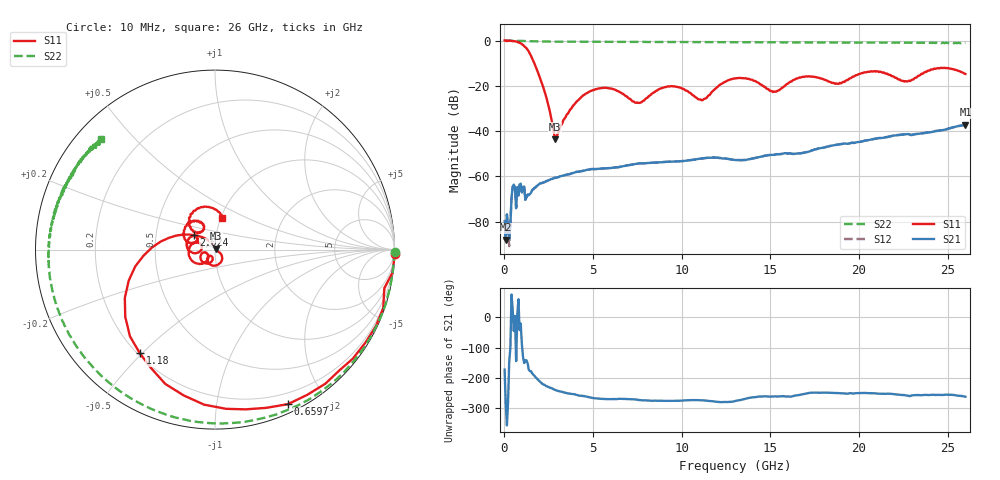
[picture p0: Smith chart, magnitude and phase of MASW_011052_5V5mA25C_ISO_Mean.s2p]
! MA-COM, USA
! Part Number: MASW-011052
! Data: 29-03-2013
! Bias Condition:
!  Isolation in OFF stage Antenna (1) to RFin (2)
!  Forward Bias (series Diode and Shunt Diode) I = 5 mA
!  Reverse Bias Voltage V = -5V
!  Temp: 25C
!  VAR RecID: Mean
# HZ S DB R 50
! F n11x n11y n21x n21y n12x n12y n22x n22y
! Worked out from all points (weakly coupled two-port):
!   401 points, 10 MHz to 26 GHz, reference 50 ohm
!   highest |S21| = -37.23 dB at 26 GHz (marker M1); lowest = -88.0 dB at 74.97 MHz (marker M2)
!   lowest |S11| = -43.6 dB at 2.869 GHz (marker M3), VSWR 1.01, Z = 50.5 + j0.437 ohm
!   |S11| at or under -10 dB: 1.683 GHz to end of sweep
!   |S22| runs from -1.2 to 0.0 dB; largest |S21 - S12| = 0.0004
!   S11 on the Smith chart (normalised r, x): 10 MHz: -11, -89; 659.8 MHz: 0.09, -1.57; 1.18 GHz: 0.21, -0.49; 2.024 GHz: 0.78, +0.13; 26 GHz: 1.02, +0.37
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1e7  0.02 -1.3  -79.88 -172.9  -88.18 -125.7  0.00 -0.8
7.4975e7  -0.03 -7.5  -87.95 74.8  -84.14 88.6  -0.01 -6.5
6.5975e8  -0.43 -64.7  -74.08 -144.9  -73.99 -143.7  -0.12 -53.0
1.1796e9  -2.93 -126.0  -70.36 -141.8  -70.37 -141.5  -0.25 -84.1
1.5694e9  -7.97 -175.2  -65.99 174.5  -66.07 173.7  -0.34 -101.1
2.0242e9  -16.98 145.2  -63.03 147.1  -62.99 146.8  -0.41 -115.9
2.8689e9  -43.63 41.2  -60.69 120.0  -60.66 120.4  -0.49 -134.5
4.3633e9  -24.79 -46.3  -57.71 100.9  -57.69 101.2  -0.54 -153.3
5.7928e9  -20.95 -101.0  -56.41 90.1  -56.41 90.2  -0.58 -164.2
7.5471e9  -27.55 -117.8  -54.34 87.4  -54.32 87.7  -0.62 -173.6
8.7167e9  -21.49 -114.7  -53.84 84.7  -53.79 85.1  -0.64 -178.2
9.7563e9  -20.49 -148.3  -53.42 84.6  -53.41 84.8  -0.67 178.0
1.1186e10  -26.29 -144.3  -52.10 85.9  -52.08 86.7  -0.69 173.5
1.3005e10  -16.76 -158.4  -52.79 83.5  -52.80 83.9  -0.74 167.8
1.5214e10  -22.55 173.2  -50.51 98.7  -50.48 99.7  -0.80 162.7
1.7358e10  -15.90 159.5  -48.48 111.0  -48.48 112.1  -0.82 157.6
1.8723e10  -18.92 153.2  -46.04 110.1  -46.01 110.8  -0.89 154.5
2.0412e10  -14.06 150.2  -44.16 109.9  -44.15 110.8  -0.92 149.9
2.1712e10  -15.19 119.6  -42.50 107.7  -42.37 109.1  -0.93 147.7
2.2621e10  -17.94 125.6  -41.45 102.2  -41.34 103.7  -0.94 145.5
2.4376e10  -12.38 121.3  -39.94 103.9  -39.92 104.9  -0.93 141.3
2.6e10  -14.78 77.0  -37.23 97.9  -37.20 99.6  -1.06 135.9
